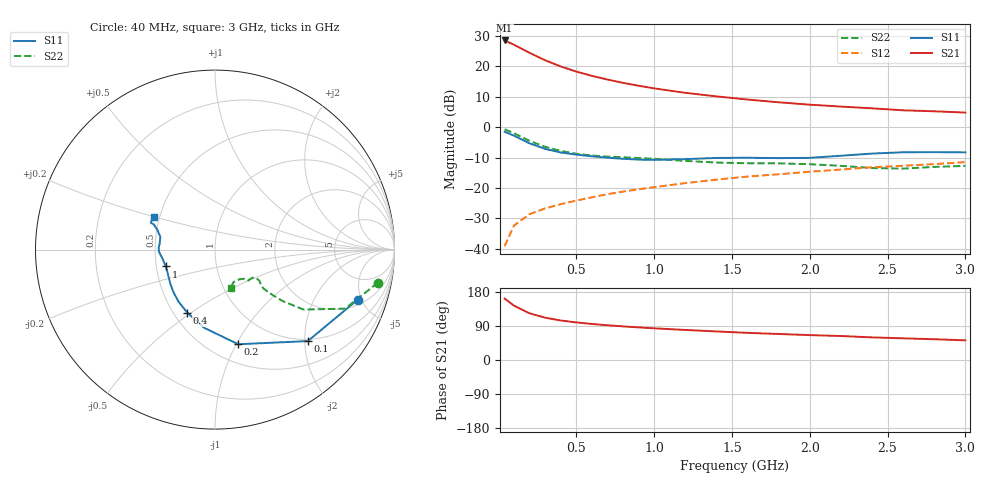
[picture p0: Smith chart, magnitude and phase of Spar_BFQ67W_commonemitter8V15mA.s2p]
! Filename:  BFQ67WJ.S2P  Version:  4.0
! NXP part #: BFQ67W  Date: Jun 1994
! Bias condition: Vce=8V, Ic=15mA
#  MHz  S  MA  R  50
! Freq  S11  S21  S12  S22  !GUM [dB]
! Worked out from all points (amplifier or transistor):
!   21 points, 40 MHz to 3 GHz, reference 50 ohm
!   highest |S21| = 28.6 dB at 40 MHz (marker M1)
!   |S21| within 3 dB of that: start of sweep to 159.9 MHz
!   unconditionally stable (mu >= 1): 757.9 MHz to end of sweep
!   at 300 MHz: K = 0.70, MSG = 24.4 dB, |S12| = -26.7 dB
!   at 1 GHz: K = 1.07, MAG = 14.7 dB, |S12| = -19.7 dB
!   at 3 GHz: K = 1.03, MAG = 7.1 dB, |S12| = -11.5 dB
!   lowest NFmin = 2.00 dB at 1 GHz
!   S11 on the Smith chart (normalised r, x): 40 MHz: 2.41, -4.64; 100 MHz: 0.96, -2.07; 200 MHz: 0.68, -1.02; 400 MHz: 0.59, -0.48; 1 GHz: 0.56, -0.12; 3 GHz: 0.47, +0.20
40  0.842 -19.4  26.81 162.2  0.011 79.0  0.926 -11.5
100  0.726 -44.6  22.82 143.4  0.024 67.7  0.796 -24.4
200  0.543 -76.2  16.78 123.2  0.037 59.9  0.596 -34.1
300  0.44 -97.9  12.67 111.7  0.046 59.3  0.476 -37.2
400  0.384 -113.7  10.01 104.3  0.054 60.3  0.407 -38.3
500  0.354 -125.1  8.254 99.2  0.062 62.1  0.366 -38.7
600  0.332 -134.1  7.01 95.1  0.07 63.6  0.342 -38.6
700  0.315 -141.7  6.095 91.7  0.079 65.1  0.328 -38.1
800  0.302 -148.4  5.381 88.7  0.087 66.5  0.32 -37.1
900  0.293 -154.8  4.82 86.1  0.095 67.4  0.311 -36.1
1000  0.29 -161.1  4.362 83.6  0.103 68.0  0.302 -35.1
1200  0.298 -171.3  3.684 79.3  0.12 69.1  0.279 -34.6
1400  0.312 -177.5  3.22 75.4  0.137 69.9  0.262 -36.7
1600  0.314 178.2  2.855 71.6  0.154 69.6  0.255 -40.4
1800  0.31 173.4  2.572 68.7  0.168 70.1  0.254 -42.6
2000  0.313 166.8  2.349 65.7  0.185 70.3  0.246 -43.0
2200  0.339 161.2  2.187 63.3  0.201 70.8  0.231 -44.6
2400  0.368 157.7  2.046 59.7  0.219 70.4  0.213 -51.3
2600  0.387 157.3  1.897 57.2  0.232 69.7  0.208 -60.2
2800  0.389 156.0  1.828 54.8  0.247 70.0  0.222 -65.3
3000  0.385 152.0  1.742 51.9  0.266 69.6  0.231 -67.7
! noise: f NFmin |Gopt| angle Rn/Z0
1000  2  0.3  77  0.289
